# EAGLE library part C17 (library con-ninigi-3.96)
NINIGI
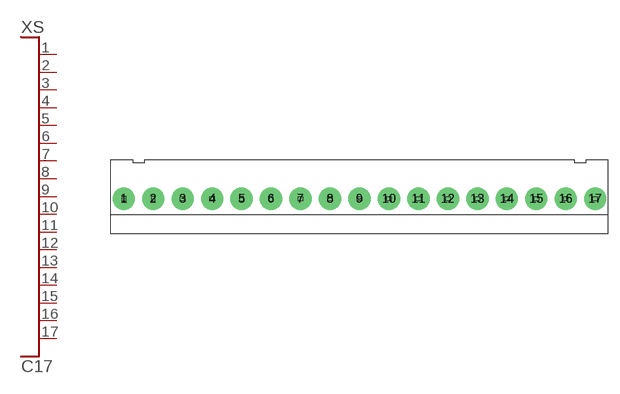
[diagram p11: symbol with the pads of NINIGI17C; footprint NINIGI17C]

Designator prefix XS

## C17  [NINIGI17C]
1  P$1
2  P$2
3  P$3
4  P$4
5  P$5
6  P$6
7  P$7
8  P$8
9  P$9
10  P$10
11  P$11
12  P$12
13  P$13
14  P$14
15  P$15
16  P$16
17  P$17

## Footprint NINIGI17C (pad centres in mm)
drill 1.6 pad 3: 1 -31.68,0; 2 -27.72,0; 3 -23.76,0; 4 -19.8,0; 5 -15.84,0; 6 -11.88,0; 7 -7.92,0; 8 -3.96,0; 9 0,0; 10 3.96,0; 11 7.92,0; 12 11.88,0; 13 15.84,0; 14 19.8,0; 15 23.76,0; 16 27.72,0; 17 31.68,0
